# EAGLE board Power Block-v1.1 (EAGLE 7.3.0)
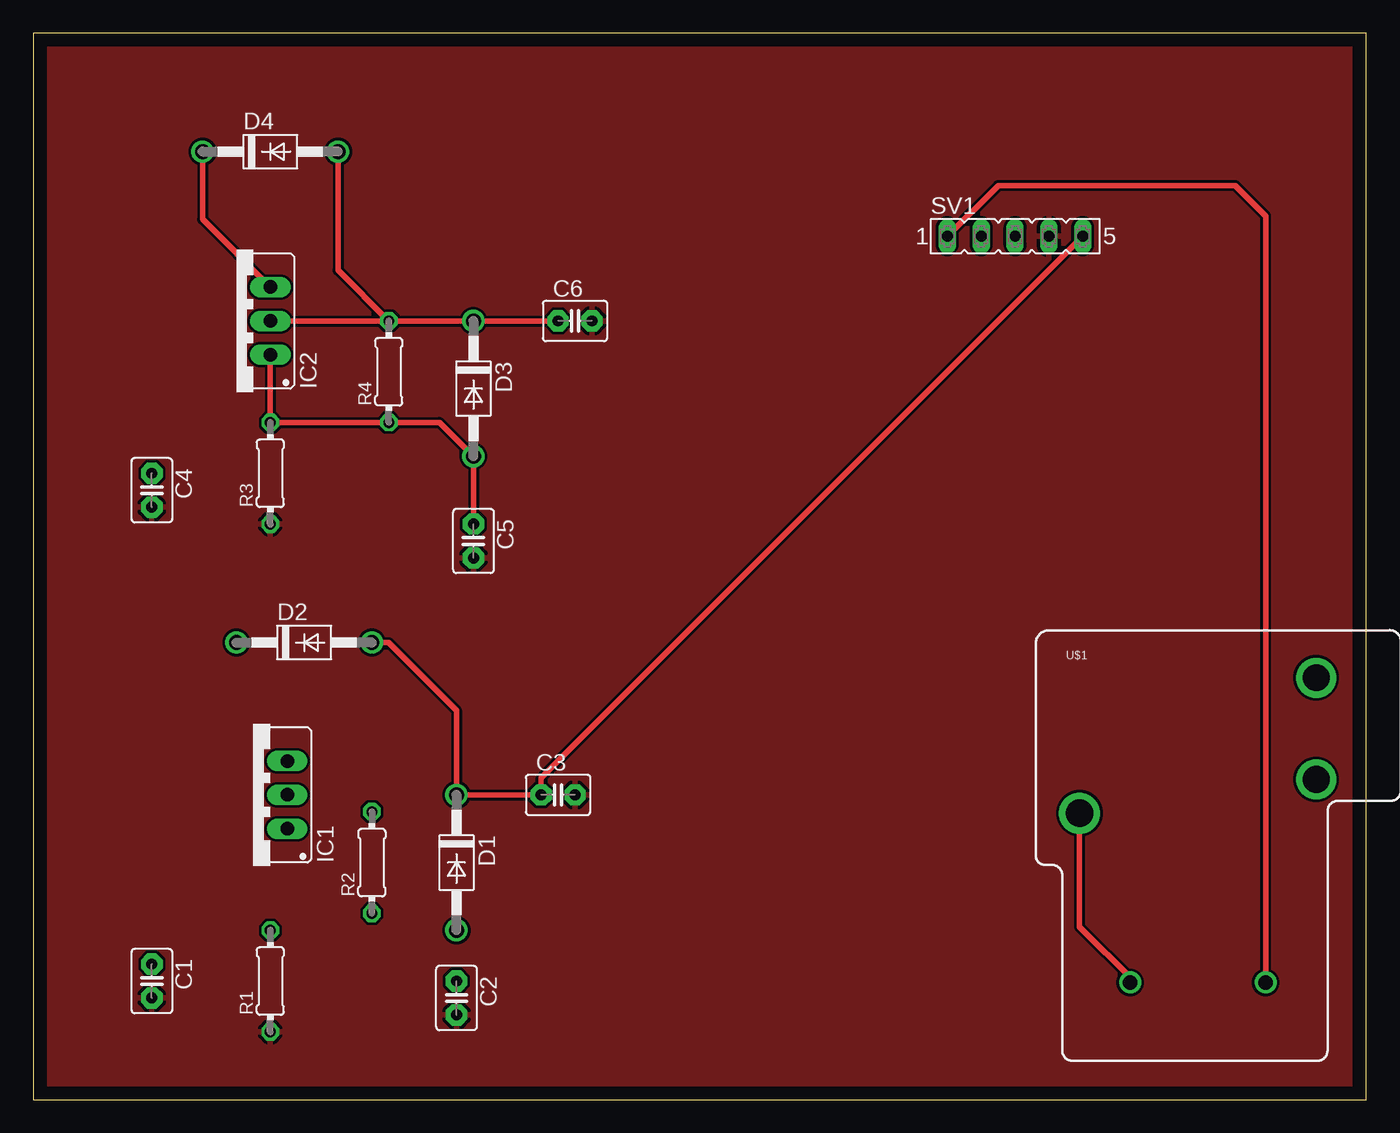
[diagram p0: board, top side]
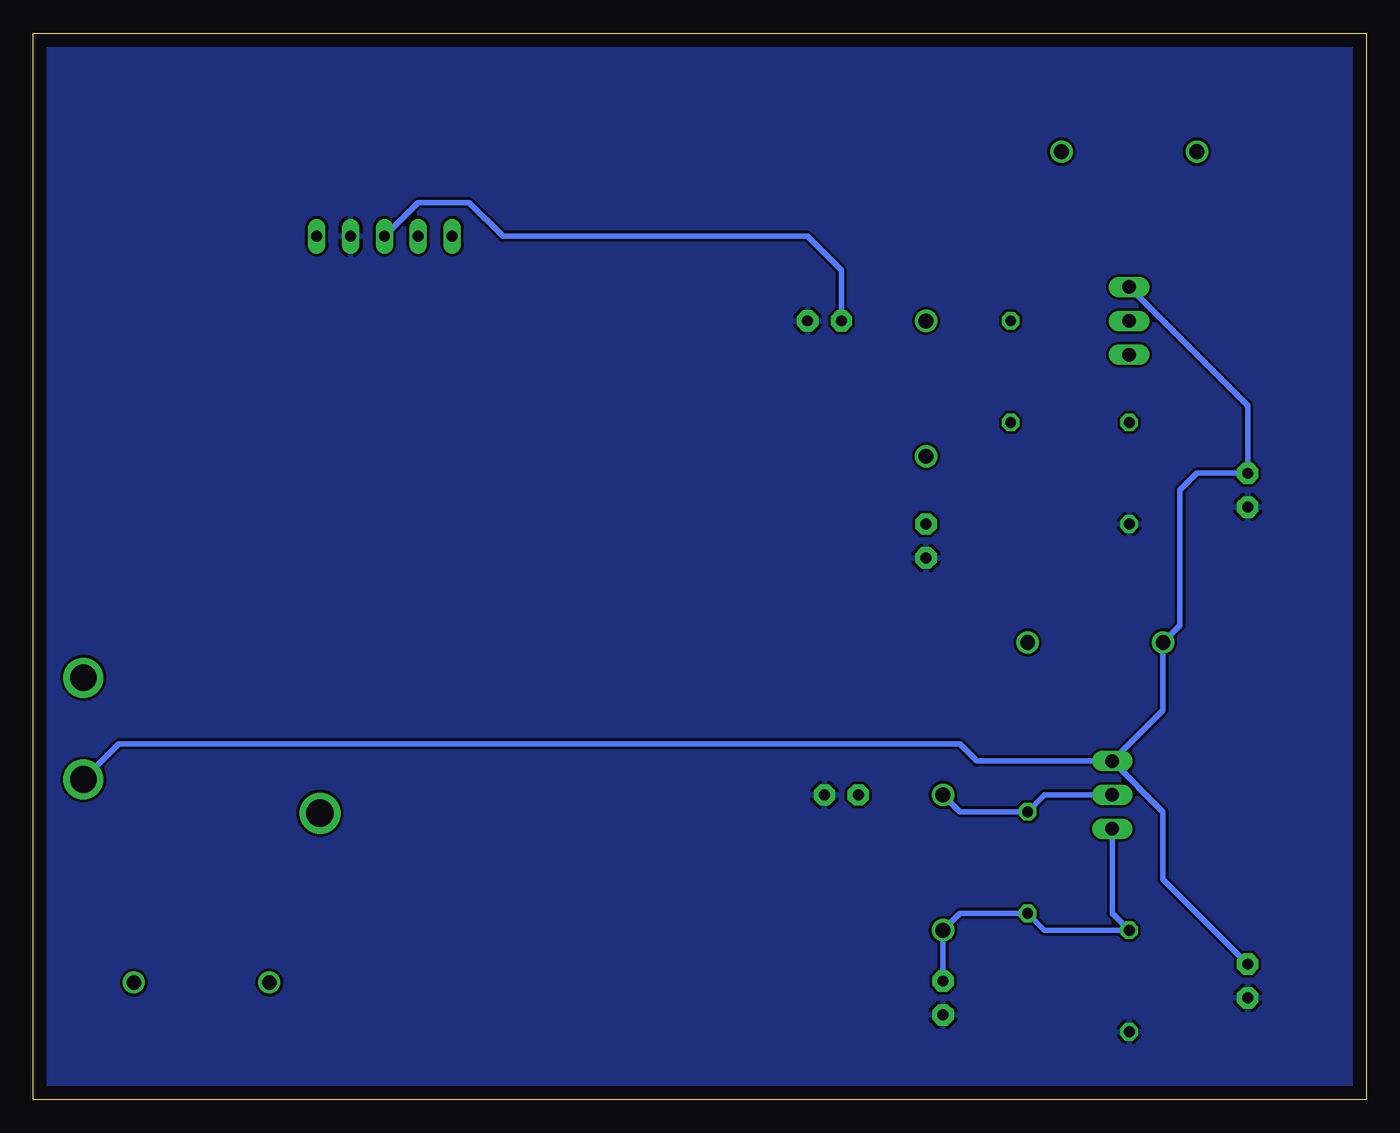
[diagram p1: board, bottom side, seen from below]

Size 100 x 80 mm. Coordinates in mm from the lower left corner, seen from the top.
Outline: 0,0 100,0 100,80 0,80 0,0
Copper layers (1*16): Top 0.035mm / dielectric 1.5mm / Bottom 0.035mm
Design rules "default": minimum track width 10mil, minimum drill 24mil, track to track 8mil, track to pad 8mil, pad to pad 8mil, via to via 8mil, smd to smd 8mil, copper to edge 40mil, drill to drill 8mil, minimum pad ring 10mil, minimum via ring 8mil, stop-mask expansion 4mil, vias tented up to drill 0mil, thermal gap 10mil

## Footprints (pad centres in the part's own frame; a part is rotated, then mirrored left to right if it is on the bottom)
C2.5-3 = drill 0.813 pad 1.6 octagon: 1 -1.27,0; 2 1.27,0
DO41-10 = drill 1.118: A 5.08,0; C -5.08,0
317TS = drill 1.016 long: 1 -2.54,-2.54; 2 0,-2.54; 3 2.54,-2.54
0204/7 = drill 0.813 octagon: 1 -3.81,0; 2 3.81,0
FE05-1 = drill 0.813 long: 1 -5.08,0; 2 -2.54,0; 3 0,0; 4 2.54,0; 5 5.08,0
RELAY-T9A-2 = drill 1.1: COIL1 -6.61,-10.27; COIL2 3.55,-10.27 | drill 2.057: MAIN -10.41,2.43 | drill 2: NC 7.35,12.6; NO 7.35,4.97

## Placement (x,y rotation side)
C1  0.1uF  [C2.5-3]  8.89,8.89 270 top
C2  1uF  [C2.5-3]  31.75,7.62 270 top
C3  1uF  [C2.5-3]  39.37,22.86 0 top
C4  0.1uF  [C2.5-3]  8.89,45.72 270 top
C5  1uF  [C2.5-3]  33.02,41.91 270 top
C6  1uF  [C2.5-3]  40.64,58.42 0 top
D1  1N4004  [DO41-10]  31.75,17.78 270 top
D2  1N4004  [DO41-10]  20.32,34.29 0 top
D3  1N4004  [DO41-10]  33.02,53.34 270 top
D4  1N4004  [DO41-10]  17.78,71.12 0 top
IC1  [317TS]  16.51,22.86 90 top
IC2  [317TS]  15.24,58.42 90 top
R1  290  [0204/7]  17.78,8.89 90 top
R2  200  [0204/7]  25.4,17.78 90 top
R3  614  [0204/7]  17.78,46.99 90 top
R4  200  [0204/7]  26.67,54.61 90 top
SV1  [FE05-1]  73.66,64.77 0 top
U$1  RELAYPTH3  [RELAY-T9A-2]  88.9,19.05 0 top

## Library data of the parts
C1-C6 = capacitor-wima
D1-D4 = diode
IC1 IC2 = v-reg
R1-R4 = rcl
SV1 = con-lsta; OC_FARNELL: unknown; OC_NEWARK: unknown
U$1 = SparkFun-Electromechanical

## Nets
+3V3: C3.1 D1.C D2.A IC1.2 R2.2 SV1.5
+5V: C6.1 D3.C D4.A IC2.2 R4.2 SV1.3
+12V: U$1.COIL1 U$1.MAIN
GND: C1.2 C2.2 C3.2 C4.2 C5.2 C6.2 R1.1 R3.1 SV1.4
N$1: C2.1 D1.A IC1.1 R1.2 R2.1
N$2: SV1.1 U$1.COIL2
N$3: C5.1 D3.A IC2.1 R3.2 R4.1
N$4: C1.1 C4.1 D2.C D4.C IC1.3 IC2.3 U$1.NO

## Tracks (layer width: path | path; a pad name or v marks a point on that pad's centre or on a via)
+3V3
  Top 0.406: D2.A 26.67,34.29 31.75,29.21 D1.C C3.1 38.1,24.13 SV1.5
  Bottom 0.406: IC1.2 24.13,22.86 R2.2 30.48,21.59 D1.C
+5V
  Top 0.406: D4.A 22.86,62.23 R4.2 | IC2.2 R4.2 | R4.2 D3.C C6.1
  Bottom 0.406: C6.1 39.37,62.23 41.91,64.77 64.77,64.77 67.31,67.31 71.12,67.31 SV1.3
+12V
  Top 0.406: U$1.MAIN 78.49,12.95 82.55,8.89 82.4,8.89 U$1.COIL1
GND
  pour Bottom: 0,80.01 0,0 100.33,0 100.33,80.01
  pour Top: 0,80.01 0,0 100.33,0 100.33,80.01
N$1
  Bottom 0.406: IC1.1 19.05,13.97 R1.2 24.13,12.7 R2.1 30.48,13.97 D1.A C2.1
N$2
  Top 0.406: U$1.COIL2 92.45,66.3 90.17,68.58 72.39,68.58 SV1.1
N$3
  Top 0.406: IC2.1 R3.2 R4.1 30.48,50.8 D3.A C5.1
N$4
  Top 0.406: D4.C 12.7,66.04 IC2.3
  Bottom 0.406: IC2.3 8.89,52.07 C4.1 12.7,46.99 13.97,45.72 13.97,35.56 D2.C 15.24,29.21 IC1.3 | IC1.3 29.21,25.4 30.48,26.67 93.6,26.67 U$1.NO | IC1.3 15.24,21.59 15.24,16.51 C1.1

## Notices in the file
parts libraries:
SparkFun-Electromechanical: Licensing: Creative Commons ShareAlike 4.0 International - https://creativecommons.org/licenses/by-sa/4.0
